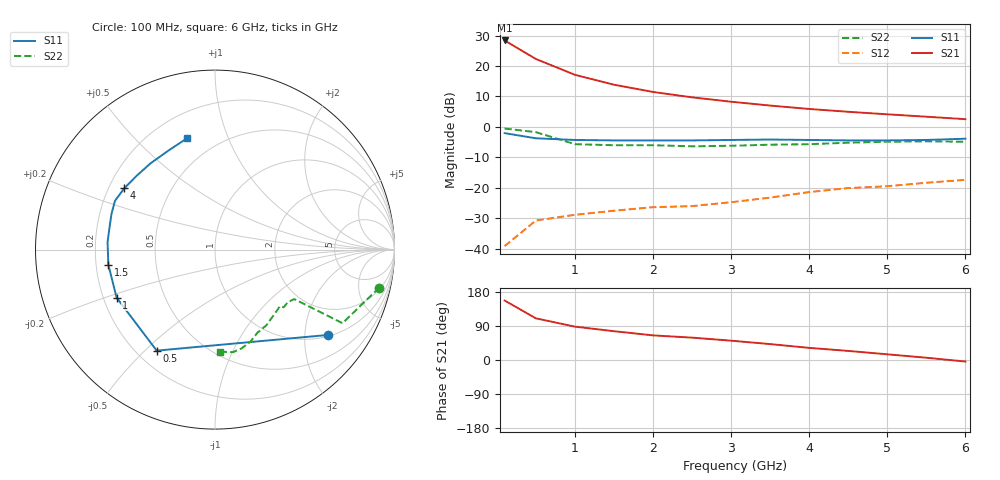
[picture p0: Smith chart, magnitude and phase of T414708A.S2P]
!AT-41470
!S-PARAMETERS at Vce=8V  Ic=10mA.  LAST UPDATED 07-21-92
# ghz s ma r 50
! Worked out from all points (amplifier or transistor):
!   13 points, 100 MHz to 6 GHz, reference 50 ohm
!   highest |S21| = 28.4 dB at 100 MHz (marker M1)
!   |S21| within 3 dB of that: start of sweep to 297.5 MHz
!   unconditionally stable (mu >= 1): 1.494 GHz to 5.188 GHz
!   at 1 GHz: K = 0.79, MSG = 23.0 dB, |S12| = -28.9 dB
!   at 3 GHz: K = 1.36, MAG = 12.9 dB, |S12| = -24.7 dB
!   at 6 GHz: K = 0.88, MSG = 10.0 dB, |S12| = -17.4 dB
!   lowest NFmin = 1.20 dB at 100 MHz
!   S11 on the Smith chart (normalised r, x): 100 MHz: 1.04, -2.62; 500 MHz: 0.28, -0.54; 1 GHz: 0.25, -0.22; 1.5 GHz: 0.25, -0.07; 4 GHz: 0.26, +0.29; 6 GHz: 0.34, +0.72
0.1  0.79 -37.0  26.27 157.0  0.011 57.0  0.94 -13.0
0.5  0.65 -120.0  13.05 110.0  0.029 40.0  0.82 -30.0
1  0.61 -154.0  7.17 88.0  0.036 41.0  0.52 -32.0
1.5  0.6 -172.0  4.93 76.0  0.042 46.0  0.5 -36.0
2  0.6 176.0  3.75 65.0  0.048 46.0  0.5 -40.0
2.5  0.6 169.0  3.06 59.0  0.05 58.0  0.48 -41.0
3  0.61 161.0  2.59 51.0  0.058 61.0  0.49 -48.0
3.5  0.62 154.0  2.24 42.0  0.069 63.0  0.51 -56.0
4  0.61 146.0  1.97 32.0  0.085 62.0  0.52 -63.0
4.5  0.6 137.0  1.77 24.0  0.099 59.0  0.55 -69.0
5  0.6 127.0  1.61 15.0  0.106 59.0  0.57 -75.0
5.5  0.61 115.0  1.47 6.0  0.121 56.0  0.58 -80.0
6  0.64 104.0  1.34 -4.0  0.135 53.0  0.57 -87.0
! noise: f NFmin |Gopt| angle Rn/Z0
0.1  1.2  0.12  5  0.17
0.5  1.2  0.11  17  0.17
1  1.3  0.06  35  0.17
2  1.6  0.21  160  0.16
4  3  0.45  -150  0.2
